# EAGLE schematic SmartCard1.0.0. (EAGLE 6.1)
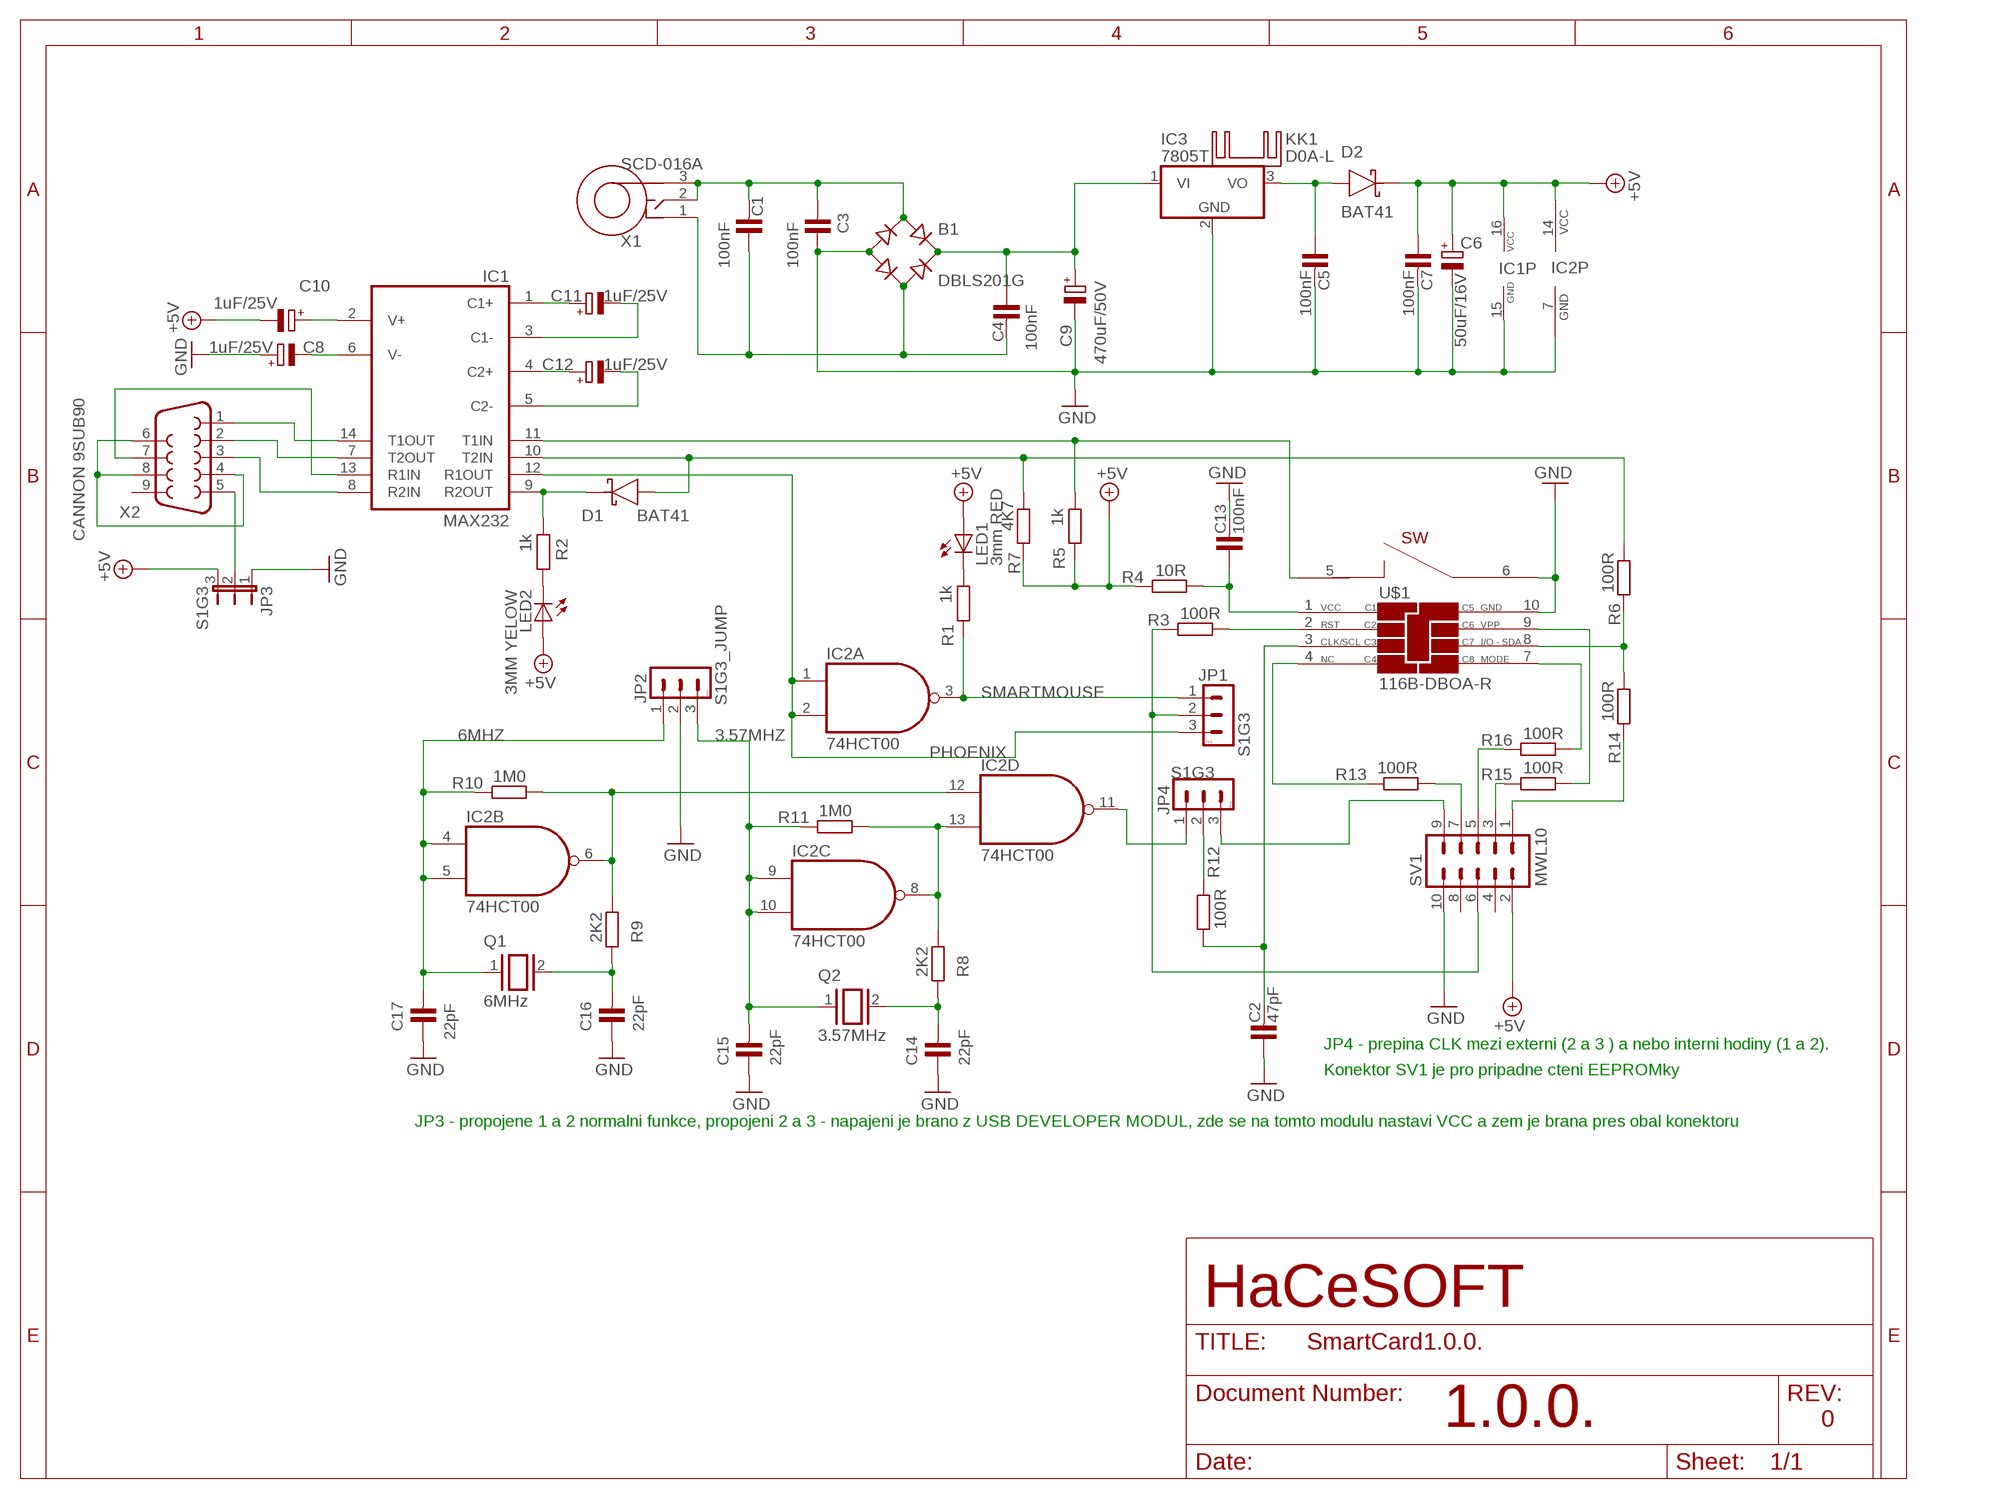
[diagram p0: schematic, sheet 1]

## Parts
B1  DBLS201G  [DBS]
C1  100nF  C-KERAMIK_2,5  [C-2,5]
C2  47pF  C-KERAMIK_2,5  [C-2,5]
C3  100nF  C-KERAMIK_2,5  [C-2,5]
C4  100nF  C-KERAMIK_2,5  [C-2,5]
C5  100nF  C-KERAMIK_2,5  [C-2,5]
C6  50uF/16V  CPOL-EUE2.5-5  [E2,5-5]
C7  100nF  C-KERAMIK_2,5  [C-2,5]
C8  1uF/25V  CPOL-EUE2.5-5  [E2,5-5]
C9  470uF/50V  CPOL-EUE3.5-10  [E3,5-10]
C10  1uF/25V  CPOL-EUE2.5-5  [E2,5-5]
C11  1uF/25V  CPOL-EUE2.5-5  [E2,5-5]
C12  1uF/25V  CPOL-EUE2.5-5  [E2,5-5]
C13  100nF  C-KERAMIK_2,5  [C-2,5]
C14  22pF  C-KERAMIK_2,5  [C-2,5]
C15  22pF  C-KERAMIK_2,5  [C-2,5]
C16  22pF  C-KERAMIK_2,5  [C-2,5]
C17  22pF  C-KERAMIK_2,5  [C-2,5]
D1  BAT41  BAT42  [DO201]
D2  BAT41  BAT42  [DO201]
IC1  MAX232  [DIL16]
IC2  74HCT00  7400D  [SO14]
IC3  7805T  [TO220H]
JP1  S1G3  S1G3_JUMP  [S1G3_JUM]
JP2  S1G3_JUMP  [S1G3_JUM]
JP3  S1G3  JP2E  [JP2]
JP4  S1G3  S1G3_JUMP  [S1G3_JUM]
KK1  D0A-L  [D02A-L]
LED1  3mm RED  LED3MM  [LED3MM]
LED2  3MM YELOW  LED3MM  [LED3MM]
Q1  6MHz  XTAL2  [Q/4]
Q2  3.57MHz  XTAL2  [Q/4]
R1  1k  R-EU_M1206  [M1206]
R2  1k  R-EU_M1206  [M1206]
R3  100R  R-EU_M1206  [M1206]
R4  10R  R-EU_M1206  [M1206]
R5  1k  R-EU_M1206  [M1206]
R6  100R  R-EU_M1206  [M1206]
R7  4K7  R-EU_M1206  [M1206]
R8  2K2  R-EU_M1206  [M1206]
R9  2K2  R-EU_M1206  [M1206]
R10  1M0  R-EU_M1206  [M1206]
R11  1M0  R-EU_M1206  [M1206]
R12  100R  R-EU_M1206  [M1206]
R13  100R  R-EU_M1206  [M1206]
R14  100R  R-EU_M1206  [M1206]
R15  100R  R-EU_M1206  [M1206]
R16  100R  R-EU_M1206  [M1206]
SV1  MWL10  ML10L  [ML10L]
U$1  116B-DBOA-R  [693030010810]
X1  SCD-016A  NAPAJECI_KONEKTOR_SCD-016A  [NAPAJECI_KONEKTOR_SCD-016A]
X2  CANNON 9SUB90  F09H  [F09H]

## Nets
3.57MHZ: C15.2 IC2.9(C:I0) IC2.10(C:I1) JP2.3 Q2.1 R11.2
6MHZ: C17.2 IC2.4(B:I0) IC2.5(B:I1) JP2.1 Q1.1 R10.2
+5V: C6.+ C7.1 C10.- D2.K IC1.16(VCC) IC2.14(P:VCC) JP3.3 LED1.A LED2.A R4.2 R5.1 R7.2 SV1.2
GND: B1.- C2.1 C3.1 C5.2 C6.- C7.2 C8.+ C9.- C13.2 C14.1 C15.1 C16.1 C17.1 IC1.15(GND) IC2.7(P:GND) IC3.2(GND) JP2.2 JP3.1 SV1.10 U$1.6(SWITCH2) U$1.10(GND)
N$1: IC1.14(T1OUT) X2.1
N$2: IC1.7(T2OUT) X2.2
N$3: IC1.8(R2IN) X2.3
N$4: X2.4 X2.6 X2.8
N$5: IC1.13(R1IN) X2.7
N$6: JP3.2 X2.5
N$7: B1.+ C4.1 C9.+ IC3.1(VI)
N$8: C10.+ IC1.2(V+)
N$9: B1.AC1 C1.2 C3.2 X1.2 X1.3(PROSTREDEK)
N$10: B1.AC2 C1.1 C4.2 X1.1(OBAL)
N$11: C5.1 D2.A IC3.3(VO)
N$12: C8.- IC1.6(V-)
N$13: C11.+ IC1.1(C1+)
N$14: C12.+ IC1.4(C2+)
N$15: C11.- IC1.3(C1-)
N$16: C12.- IC1.5(C2-)
N$17: LED1.K(C) R1.2
N$18: D1.K IC1.9(R2OUT) R2.2
N$19: D1.A IC1.10(T2IN) R6.1 R7.1
N$20: LED2.K(C) R2.1
N$21: JP1.2 R3.2 SV1.6
N$22: R3.1 U$1.2(RST)
N$23: C13.1 R4.1 U$1.1(VCC)
N$24: R6.2 R14.1 U$1.8(I/O-SDA)
N$25: IC1.11(T1IN) R5.2 U$1.5(SWITCH1)
N$26: IC2.11(D:O) JP4.1
N$27: IC2.6(B:O) IC2.12(D:I0) R9.1 R10.1
N$28: C16.2 Q1.2 R9.2
N$29: C2.2 R12.1 U$1.3(CLK/SCL)
N$30: IC2.8(C:O) IC2.13(D:I1) R8.1 R11.1
N$31: C14.2 Q2.2 R8.2
N$32: JP4.3 SV1.9
N$33: JP4.2 R12.2
N$35: R13.1 SV1.7
N$36: R13.2 U$1.4(NC)
N$37: R14.2 SV1.1
N$38: R15.1 U$1.9(VPP)
N$39: R16.1 U$1.7(MODE)
N$40: R15.2 SV1.3
N$41: R16.2 SV1.5
PHOENIX: IC1.12(R1OUT) IC2.1(A:I0) IC2.2(A:I1) JP1.3
SMARTMOUSE: IC2.3(A:O) JP1.1 R1.1
Unconnected: Q1.SHILED@1(SHILED_OSC) Q1.SHILED@2(SHILED_OSC) Q2.SHILED@1(SHILED_OSC) Q2.SHILED@2(SHILED_OSC) SV1.4 SV1.8 X2.9

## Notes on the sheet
- JP4 - prepina CLK mezi externi (2 a 3 ) a nebo interni hodiny (1 a 2).
- Konektor SV1 je pro pripadne cteni EEPROMky
- JP3 - propojene 1 a 2 normalni funkce, propojeni 2 a 3 - napajeni je brano z USB DEVELOPER MODUL, zde se na tomto modulu nastavi VCC a zem je brana pres obal konektoru
- HaCeSOFT
- 1.0.0. | 0

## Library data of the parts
B1 = rectifier:DB?*G: Single Phase 1.0 AMP Glass Passivated Bridge Rectifier Taiwan Semiconductor Co.,Ltd. - TSC Source: http://www.taiwansemi.com/TSCbig5/ezcatfiles/cust/img/img/db101g.pdf http://www.ts.com.tw/db/pictures/modules/PDT/PDT060207001/DBLS201G.pdf
C1-C5 C7 C13-C17 = #hacesoft:C-KERAMIK: Kondenzator - keramicky
C6 C8-C12 = rcl:CPOL-EU: POLARIZED CAPACITOR, European symbol
D1 D2 = #_GM99:BAT42
IC1 = maxim:MAX232: RS232 TRANSEIVER; MF: MAXIM; MPN: MAX232ACPE+; OC_FARNELL: 9723773; OC_NEWARK: 68K4544
IC2 = 74xx-us:74*00: Quad 2-input NAND gate
IC3 = linear:78*: Positive VOLTAGE REGULATOR Source: http://cache.national.com/ds/LM/LM78L05.pdf http://www.fairchildsemi.com/ds/LM/LM7805.pdf
JP1 JP2 JP4 = #PaJa_konektory:S1G3_JUMP: Radove konektory - koliky - 3x
JP3 = #hacesoft:JP2E: JUMPER
KK1 = heatsink:D0A-L: HEATSINK
LED1 LED2 = led:LED: LED
Q1 Q2 = #hacesoft:XTAL: CRYSTAL
R1-R16 = resistor:R-EU_: RESISTOR, European symbol
SV1 = con-ml:ML10L: HARTING; OC_FARNELL: unknown; OC_NEWARK: unknown
U$1 = Smart Card Socket Through Hole Type, Single Port:116B-DBOA-R
X1 = #hacesoft:NAPAJECI_KONEKTOR_SCD-016A
X2 = con-subd:F09: SUB-D; OC_FARNELL: unknown; OC_NEWARK: unknown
